(* Logix 5000 AddOnInstructionDefinition export NORD_VFDcontrol_ON_Inst100_101; software revision 24.02 *)

TYPE FI_Data_IN :
STRUCT
   ConnectionFaulted : BOOL;
   RunMode : BOOL;
   Data : INT[6];   // Actual Values
END_STRUCT
END_TYPE

TYPE FI_Data_OUT :
STRUCT
   Data : INT[6];   // Control Data
END_STRUCT
END_TYPE

ADD_ON_INSTRUCTION NORD_VFDcontrol_ON_Inst100_101   (* revision 1.1, vendor NORD Drivesystems, ExecutePrescan *)
// Control Block for NORD SK 3xxP VFD
// Revision note:
// Rev 1.1
// Better Ready Start Condition Logic
// Added Inhibited Output
// Added Fault Active Output
// Rev 1.0Connection to SK3xxP
// Instances: Output 100/Input 101
// For VFD Series:
//    - ON (SK 300P Series)
VAR_IN_OUT
   FI_Status : _0342:SK300P_DE5BFA94:I:0; {required}   // Input Data Map of VFD
   FI_Control : _0342:SK300P_E8E6FFA2:O:0; {required}   // Output Data Map of VFD
END_VAR
VAR_INPUT
   VFD_Number : SINT := 1;   // Number of VFD to control (1 for Instance 100/101)
   EnableFwd : BOOL; {visible}   // HIGH = Enable CW
   EnableRev : BOOL; {visible}   // HIGH = Enable CCW
   DisableVoltage : BOOL := 1; {visible}   // LOW = No Output Voltage
   QuickStop : BOOL := 1; {visible}   // LOW = Emergency Stop Active
   FaultAckn : BOOL; {visible}   // Error / Fault Acknowledgement on Rising Edge
   ParameterSet : SINT := 1; {visible}   // Parameter Set Range 1-4, If less than 1 or greater than 4, set to default of 1
   Activate32BitSetpoint2_3 : BOOL; {visible}   // HIGH = Activate 32Bit Setpoint combining Setpoint 2 & 3
   Activate32BitSetpoint4_5 : BOOL; {visible}
   ControlWordBit8_P480_11 : BOOL; {visible}   // Control Word Bit 8 Function set in P480[11]
   ControlWordBit9_P480_12 : BOOL; {visible}   // Control Word Bit 9 Function set in P480[12]
   ControlWord : ALIAS FOR Control_Word; {access None, visible}   // Control Word Read Only Version
   Setpoint1 : INT; {visible}   // Setpoint 1 Function set in P546[1]
   Setpoint2 : INT; {visible}   // Setpoint 2 Function set in P546[2], deactivated if "PositioningActiveBitt" is set
   Setpoint3 : INT; {visible}   // Setpoint 3 Function set in P546[3], deactivated if "PositioningActiveBitt" is set
   Setpoint4 : INT; {visible}   // Setpoint 4 Reserved
   Setpoint5 : INT; {visible}   // Setpoint 5 Reserved
   Setpoint2_3_32bit : DINT; {visible}   // 32 Bit Setpoint 2 & 3 combined for positioning
   Setpoint4_5_32bit : DINT; {visible}   // 32 Bit Setpoint 4 & 5 combined for positioning
END_VAR
VAR_OUTPUT
   StatusWord : INT; {access Read Only, visible}   // Status Word
        .0   // Ready to Start
        .1   // Ready for Operation
        .2   // Operation Enabled
        .3   // Fault
        .4   // Voltage Enabled
        .5   // No Emergency Stop
        .6   // Starting Disabled
        .7   // Warning Active
        .8   // Setpoint Reached
        .9   // Bus Controller Active
        .10   // Function P481[9]
        .11   // Rotation Right Active
        .12   // Rotation Left Active
        .13   // Function P481[10]
        .14   // Parameter Set Bit 0
        .15   // Parameter Set Bit 1
   ActiveParameterSet : SINT; {access Read Only, visible}   // Displays active parameter set
   CommunicationOK : BOOL; {access Read Only, visible}   // HIGH = Communication is OK
   ReadyToStart : BOOL; {access Read Only, visible}   // HIGH = Drive Ready to Start
   VFD_Enabled : BOOL; {access Read Only, visible}   // HIGH = VFD is Enabled
   Inhibited : BOOL; {access Read Only, visible}   // VFD is Inhibited
   Warning : BOOL; {access Read Only, visible}   // HIGH = Drive has a Warning
   Faulted : BOOL; {access Read Only, visible}   // HIGH = Drive Faulted
   FaultActive : BOOL; {access Read Only, visible}   // Fault Conditions are Currently Active
   StatusWordBit10_P481_9 : BOOL; {access Read Only, visible}   // Status Word Bit 10 Function set in P481[09]
   StatusWordBit13_P481_10 : BOOL; {access Read Only, visible}   // Status Word Bit 13 Function set in P481[10]
   ActualValue1 : INT; {access Read Only, visible}   // Actual Value 1 Function set in P543[1]
   ActualValue2 : INT; {access Read Only, visible}   // Actual Value 2 Function set in P543[2]
   ActualValue3 : INT; {access Read Only, visible}   // Actual Value 3 Function set in P543[3]
   ActualValue4 : INT; {access Read Only, visible}   // Actual Value 4 Reserved
   ActualValue5 : INT; {access Read Only, visible}   // Actual Value 5 Reserved
   ActualValue2_3_32bit : DINT; {access Read Only, visible}   // 32 Bit Actual Value 2 & 3 Combined for Positioning
   ActualValue4_5_32bit : DINT; {access Read Only, visible}   // 32 Bit Actual Value 4 & 5 Combined for Positioning
END_VAR
VAR
   Index : INT; {access None}   // Index of process data based on VFD_Number
   Control_Word : INT; {access None}   // Control Word
        .0   // Enable Operation
        .1   // Disable Voltage (Low level disables the output voltage of the drive and stops the VFD)
        .2   // Emergency Stop (Low level activates QuickStop mode and stops the VFD)
        .3   // Ready for Operation
        .4   // Enable Pulses
        .5   // Enable Ramp
        .6   // Enable Setpoint
        .7   // Error Acknowledge
        .8   // Function P480[11]
        .9   // Function P480[12]
        .10   // Control Data Valid
        .11   // Rotation Direction Clockwise
        .12   // Rotation Direction Counter-Clockwise
        .13   // Reserved
        .14   // Parameter Set Bit 0
        .15   // Parameter Set Bit 1
   Control : FI_Data_OUT; {access None}
   Status : FI_Data_IN; {access None}
   LowWordOf32BitSetpoint2_3 : DINT; {access None}
   Temporary_Variable_32BitSepoint2_3 : DINT; {access None}
   HighWordOf32BitSetpoint2_3 : DINT; {access None}
   Temporary_Variable_32BitSepoint4_5 : DINT; {access None}
   HighWordOf32BitSetpoint4_5 : DINT; {access None}
   LowWordOf32BitSetpoint4_5 : DINT; {access None}
END_VAR

ROUTINE Logic   (* ladder *)
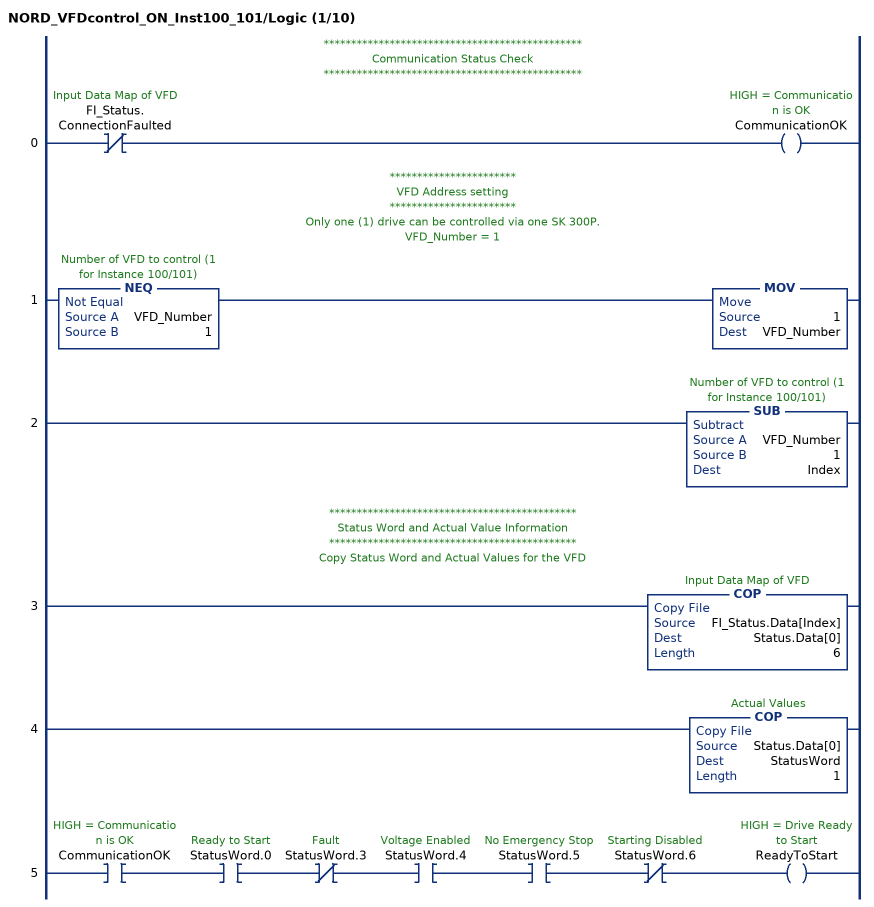
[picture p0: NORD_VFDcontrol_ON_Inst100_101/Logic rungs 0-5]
   // ***********************************************
   // Communication Status Check
   // ***********************************************
   0: XIO(FI_Status.ConnectionFaulted)OTE(CommunicationOK);
   // ***********************
   // VFD Address setting
   // ***********************
   // Only one (1) drive can be controlled via one SK 300P.
   // VFD_Number = 1
   1: NEQ(VFD_Number,1)MOV(1,VFD_Number);
   2: SUB(VFD_Number,1,Index);
   // *********************************************
   // Status Word and Actual Value Information
   // *********************************************
   // Copy Status Word and Actual Values for the VFD
   3: COP(FI_Status.Data[Index],Status.Data[0],6);
   4: COP(Status.Data[0],StatusWord,1);
   5: XIC(CommunicationOK)XIC(StatusWord.0)XIO(StatusWord.3)XIC(StatusWord.4)XIC(StatusWord.5)XIO(StatusWord.6)OTE(ReadyToStart);
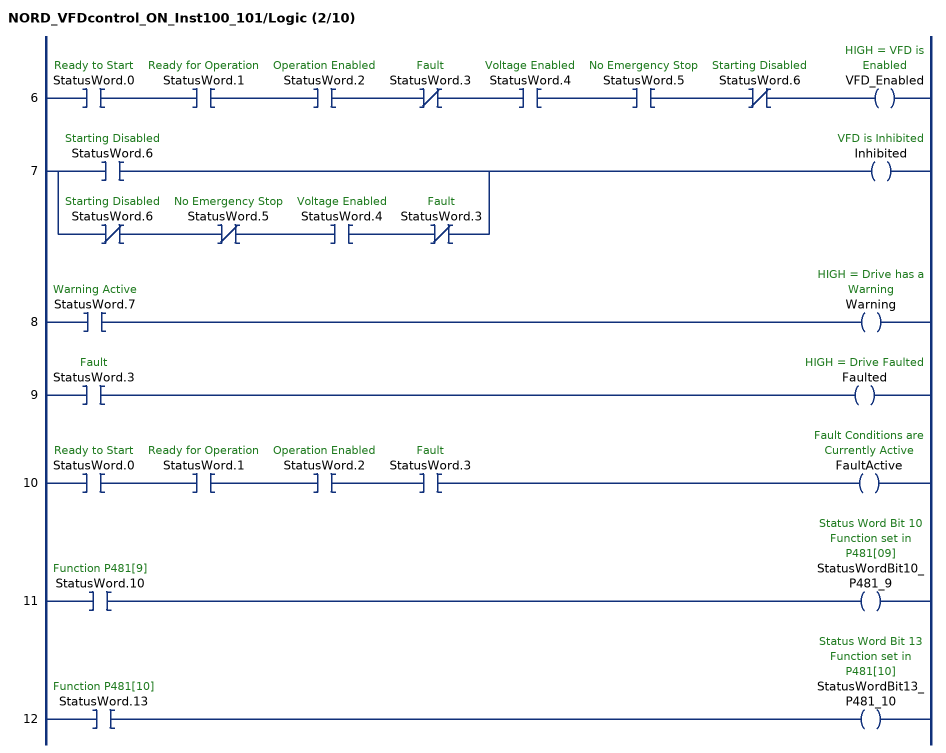
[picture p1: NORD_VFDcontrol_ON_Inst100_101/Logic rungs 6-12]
   6: XIC(StatusWord.0)XIC(StatusWord.1)XIC(StatusWord.2)XIO(StatusWord.3)XIC(StatusWord.4)XIC(StatusWord.5)XIO(StatusWord.6)OTE(VFD_Enabled);
   7: [XIC(StatusWord.6) ,XIO(StatusWord.6) XIO(StatusWord.5) XIC(StatusWord.4) XIO(StatusWord.3) ]OTE(Inhibited);
   8: XIC(StatusWord.7)OTE(Warning);
   9: XIC(StatusWord.3)OTE(Faulted);
   10: XIC(StatusWord.0)XIC(StatusWord.1)XIC(StatusWord.2)XIC(StatusWord.3)OTE(FaultActive);
   11: XIC(StatusWord.10)OTE(StatusWordBit10_P481_9);
   12: XIC(StatusWord.13)OTE(StatusWordBit13_P481_10);
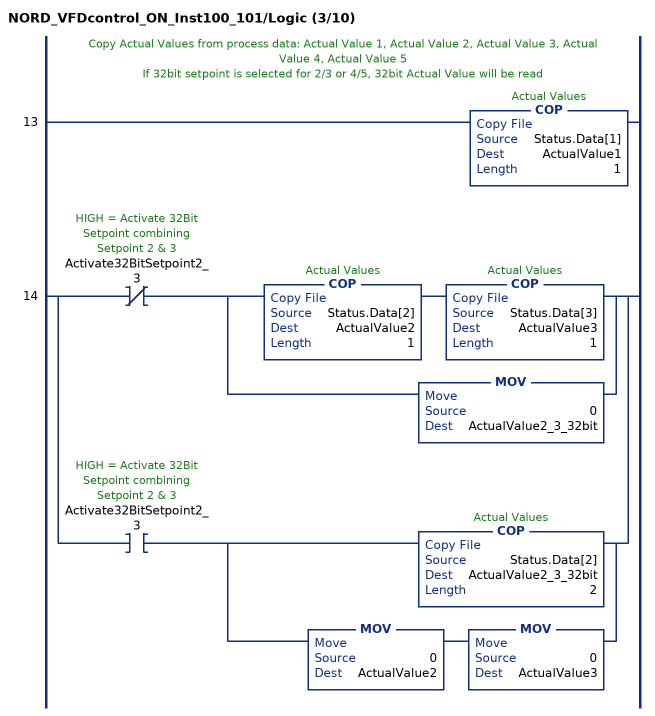
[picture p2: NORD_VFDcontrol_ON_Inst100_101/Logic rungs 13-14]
   // Copy Actual Values from process data: Actual Value 1, Actual Value 2, Actual Value 3, Actual Value 4, Actual Value 5
   // If 32bit setpoint is selected for 2/3 or 4/5, 32bit Actual Value will be read
   13: COP(Status.Data[1],ActualValue1,1);
   14: [XIO(Activate32BitSetpoint2_3) [COP(Status.Data[2],ActualValue2,1) COP(Status.Data[3],ActualValue3,1) ,MOV(0,ActualValue2_3_32bit) ] ,XIC(Activate32BitSetpoint2_3) [COP(Status.Data[2],ActualValue2_3_32bit,2) ,MOV(0,ActualValue2) MOV(0,ActualValue3) ] ];
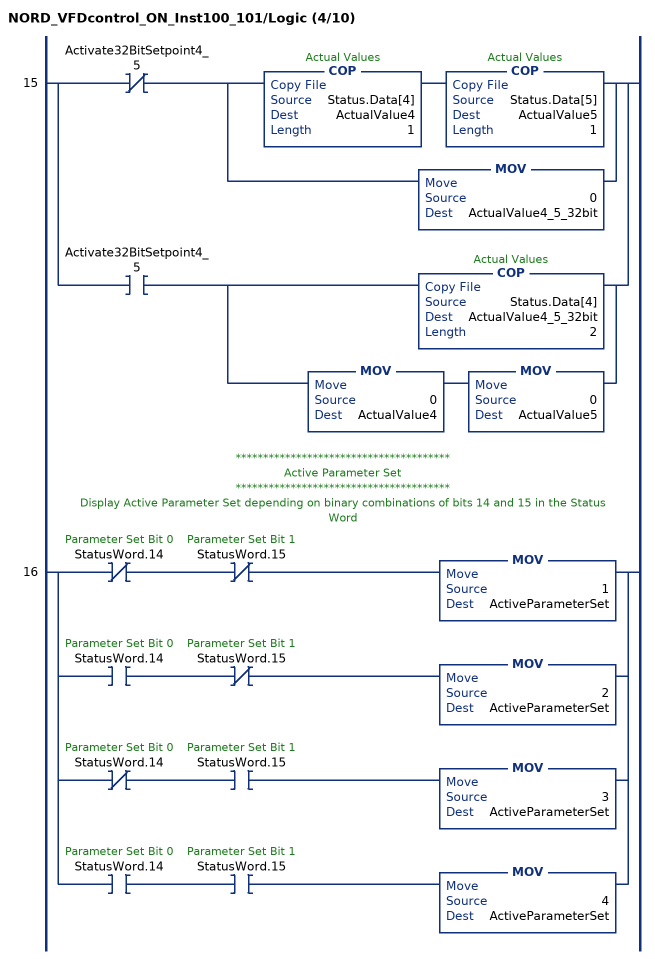
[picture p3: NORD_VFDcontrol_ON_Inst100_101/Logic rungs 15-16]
   15: [XIO(Activate32BitSetpoint4_5) [COP(Status.Data[4],ActualValue4,1) COP(Status.Data[5],ActualValue5,1) ,MOV(0,ActualValue4_5_32bit) ] ,XIC(Activate32BitSetpoint4_5) [COP(Status.Data[4],ActualValue4_5_32bit,2) ,MOV(0,ActualValue4) MOV(0,ActualValue5) ] ];
   // ***************************************
   // Active Parameter Set
   // ***************************************
   // Display Active Parameter Set depending on binary combinations of bits 14 and 15 in the Status Word
   16: [XIO(StatusWord.14) XIO(StatusWord.15) MOV(1,ActiveParameterSet) ,XIC(StatusWord.14) XIO(StatusWord.15) MOV(2,ActiveParameterSet) ,XIO(StatusWord.14) XIC(StatusWord.15) MOV(3,ActiveParameterSet) ,XIC(StatusWord.14) XIC(StatusWord.15) MOV(4,ActiveParameterSet) ];
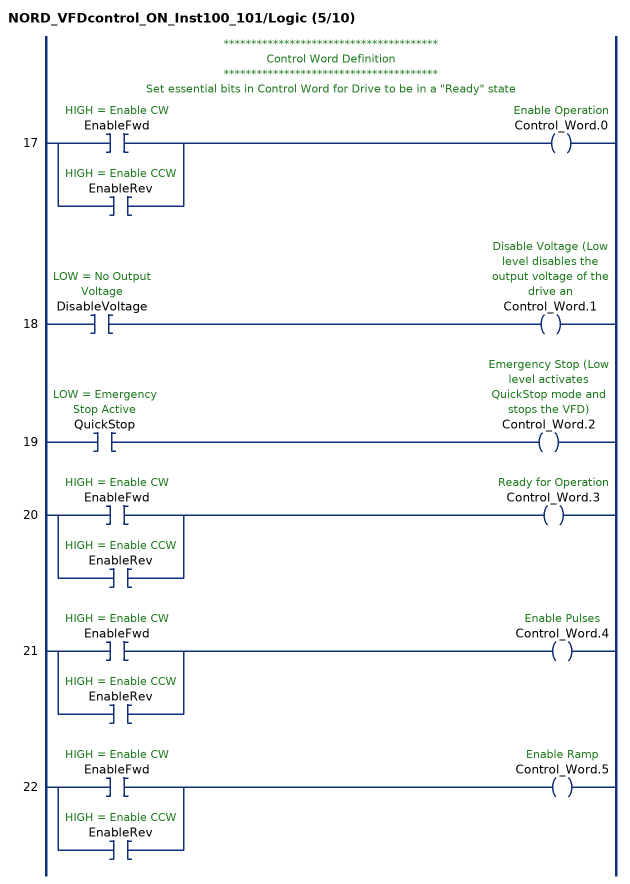
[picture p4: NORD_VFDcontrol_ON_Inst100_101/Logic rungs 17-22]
   // ***************************************
   // Control Word Definition
   // ***************************************
   // Set essential bits in Control Word for Drive to be in a "Ready" state
   17: [XIC(EnableFwd) ,XIC(EnableRev) ]OTE(Control_Word.0);
   18: XIC(DisableVoltage)OTE(Control_Word.1);
   19: XIC(QuickStop)OTE(Control_Word.2);
   20: [XIC(EnableFwd) ,XIC(EnableRev) ]OTE(Control_Word.3);
   21: [XIC(EnableFwd) ,XIC(EnableRev) ]OTE(Control_Word.4);
   22: [XIC(EnableFwd) ,XIC(EnableRev) ]OTE(Control_Word.5);
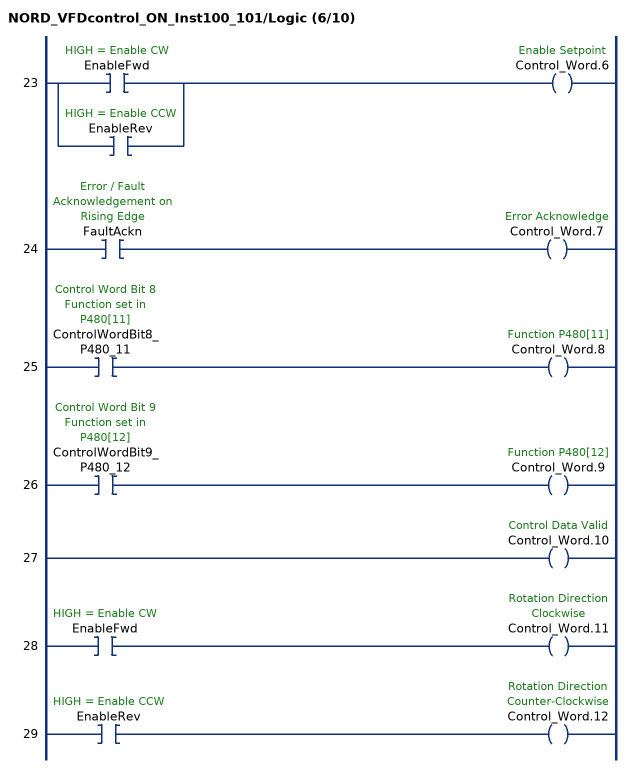
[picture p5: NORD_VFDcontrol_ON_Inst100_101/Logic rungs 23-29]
   23: [XIC(EnableFwd) ,XIC(EnableRev) ]OTE(Control_Word.6);
   24: XIC(FaultAckn)OTE(Control_Word.7);
   25: XIC(ControlWordBit8_P480_11)OTE(Control_Word.8);
   26: XIC(ControlWordBit9_P480_12)OTE(Control_Word.9);
   27: OTE(Control_Word.10);
   28: XIC(EnableFwd)OTE(Control_Word.11);
   29: XIC(EnableRev)OTE(Control_Word.12);
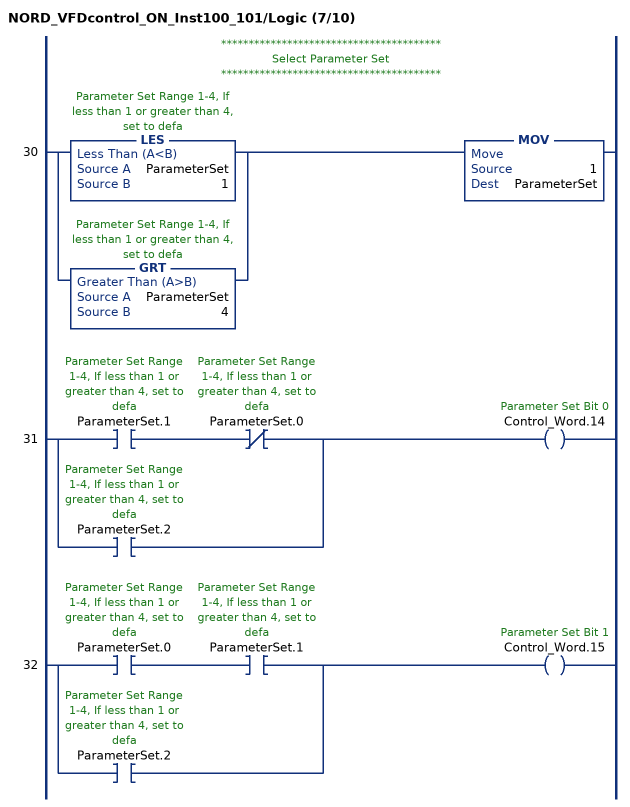
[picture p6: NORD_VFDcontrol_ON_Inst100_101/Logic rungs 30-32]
   // ****************************************
   // Select Parameter Set
   // ****************************************
   30: [LES(ParameterSet,1) ,GRT(ParameterSet,4) ]MOV(1,ParameterSet);
   31: [XIC(ParameterSet.1) XIO(ParameterSet.0) ,XIC(ParameterSet.2) ]OTE(Control_Word.14);
   32: [XIC(ParameterSet.0) XIC(ParameterSet.1) ,XIC(ParameterSet.2) ]OTE(Control_Word.15);
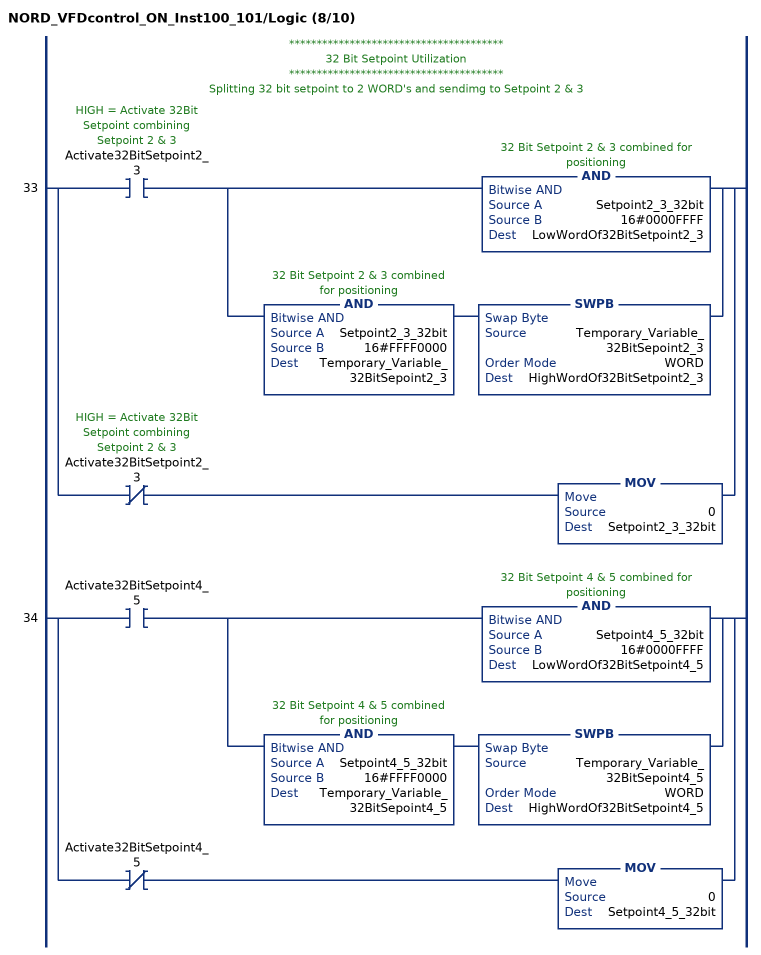
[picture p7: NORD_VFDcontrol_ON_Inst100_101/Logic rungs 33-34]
   // ***************************************
   // 32 Bit Setpoint Utilization
   // ***************************************
   // Splitting 32 bit setpoint to 2 WORD's and sendimg to Setpoint 2 & 3
   33: [XIC(Activate32BitSetpoint2_3) [AND(Setpoint2_3_32bit,16#0000FFFF,LowWordOf32BitSetpoint2_3) ,AND(Setpoint2_3_32bit,16#FFFF0000,Temporary_Variable_32BitSepoint2_3) SWPB(Temporary_Variable_32BitSepoint2_3,WORD,HighWordOf32BitSetpoint2_3) ] ,XIO(Activate32BitSetpoint2_3) MOV(0,Setpoint2_3_32bit) ];
   34: [XIC(Activate32BitSetpoint4_5) [AND(Setpoint4_5_32bit,16#0000FFFF,LowWordOf32BitSetpoint4_5) ,AND(Setpoint4_5_32bit,16#FFFF0000,Temporary_Variable_32BitSepoint4_5) SWPB(Temporary_Variable_32BitSepoint4_5,WORD,HighWordOf32BitSetpoint4_5) ] ,XIO(Activate32BitSetpoint4_5) MOV(0,Setpoint4_5_32bit) ];
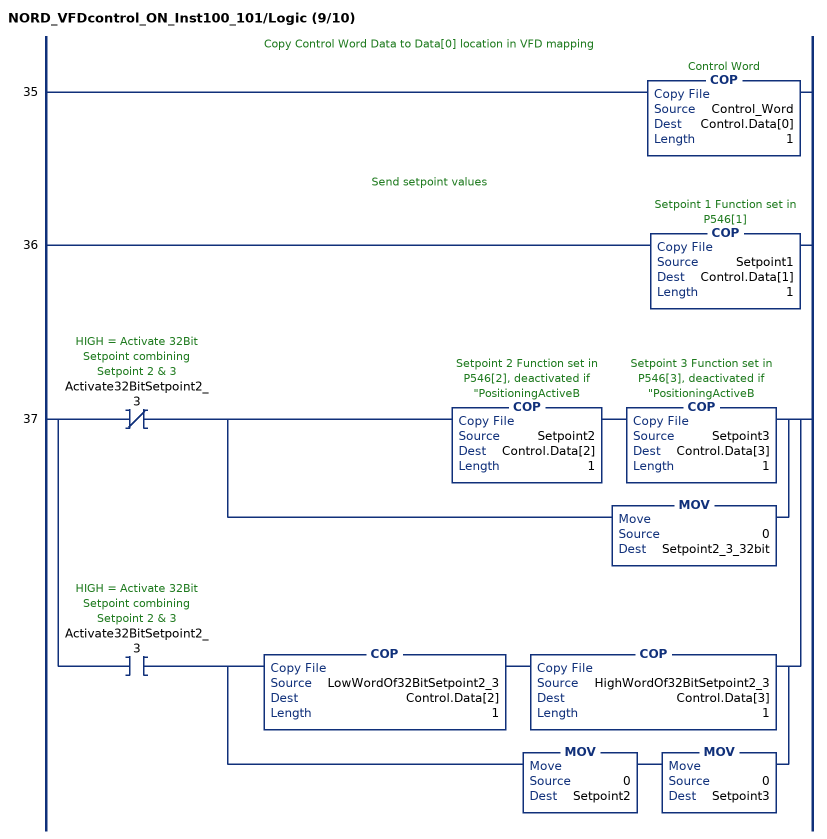
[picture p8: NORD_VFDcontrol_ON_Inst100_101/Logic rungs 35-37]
   // Copy Control Word Data to Data[0] location in VFD mapping
   35: COP(Control_Word,Control.Data[0],1);
   // Send setpoint values
   36: COP(Setpoint1,Control.Data[1],1);
   37: [XIO(Activate32BitSetpoint2_3) [COP(Setpoint2,Control.Data[2],1) COP(Setpoint3,Control.Data[3],1) ,MOV(0,Setpoint2_3_32bit) ] ,XIC(Activate32BitSetpoint2_3) [COP(LowWordOf32BitSetpoint2_3,Control.Data[2],1) COP(HighWordOf32BitSetpoint2_3,Control.Data[3],1) ,MOV(0,Setpoint2) MOV(0,Setpoint3) ] ];
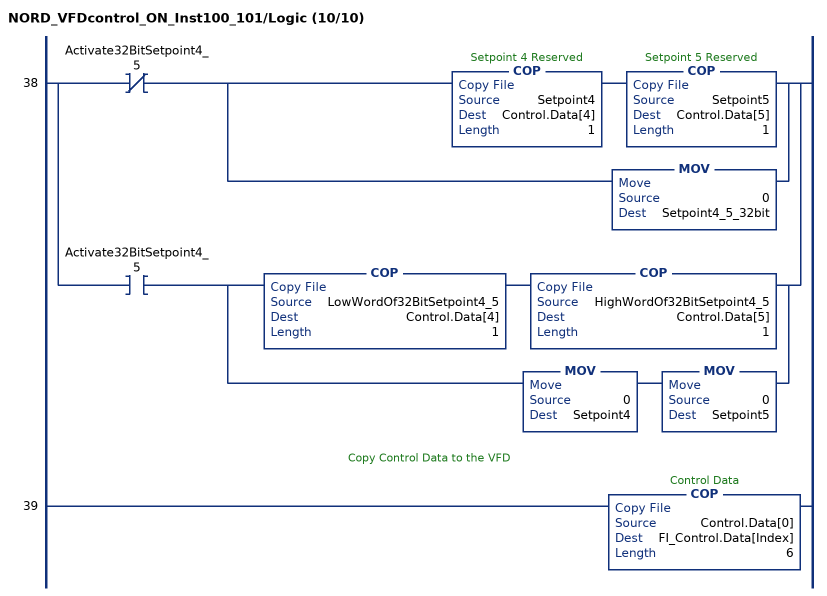
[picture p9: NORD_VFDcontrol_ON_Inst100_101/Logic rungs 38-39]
   38: [XIO(Activate32BitSetpoint4_5) [COP(Setpoint4,Control.Data[4],1) COP(Setpoint5,Control.Data[5],1) ,MOV(0,Setpoint4_5_32bit) ] ,XIC(Activate32BitSetpoint4_5) [COP(LowWordOf32BitSetpoint4_5,Control.Data[4],1) COP(HighWordOf32BitSetpoint4_5,Control.Data[5],1) ,MOV(0,Setpoint4) MOV(0,Setpoint5) ] ];
   // Copy Control Data to the VFD
   39: COP(Control.Data[0],FI_Control.Data[Index],6);
END_ROUTINE

ROUTINE Prescan   (* ladder *)
// Executed prior to first scan of AOI
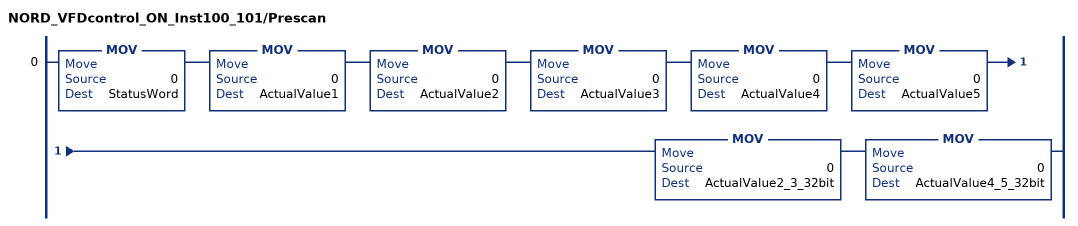
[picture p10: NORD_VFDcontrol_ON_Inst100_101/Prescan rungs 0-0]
   0: MOV(0,StatusWord)MOV(0,ActualValue1)MOV(0,ActualValue2)MOV(0,ActualValue3)MOV(0,ActualValue4)MOV(0,ActualValue5)MOV(0,ActualValue2_3_32bit)MOV(0,ActualValue4_5_32bit);
END_ROUTINE
END_ADD_ON_INSTRUCTION
